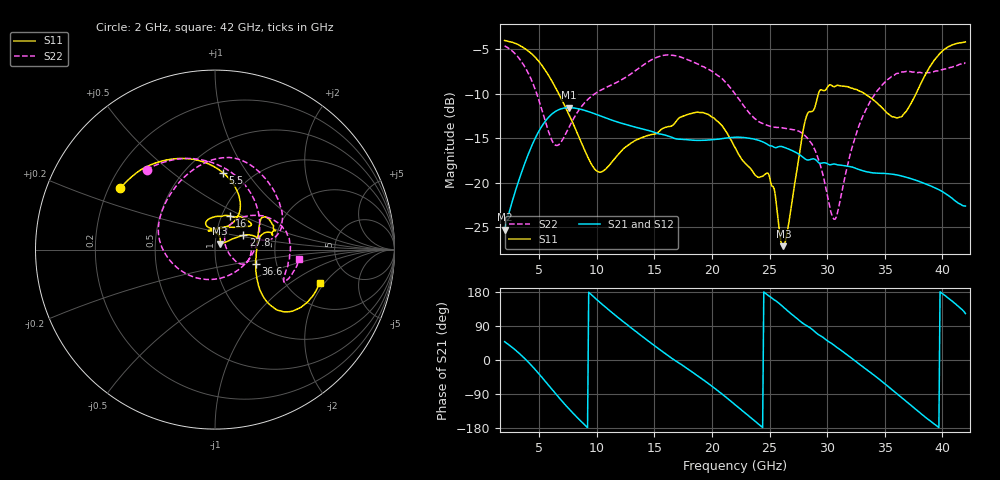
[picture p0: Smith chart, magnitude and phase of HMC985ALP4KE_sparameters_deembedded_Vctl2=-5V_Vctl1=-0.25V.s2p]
!s2p File: Measurements: S11, S21, S12, S22
# GHz S dB R 50.0
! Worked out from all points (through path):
!   401 points, 2 GHz to 42 GHz, reference 50 ohm
!   highest |S21| = -11.58 dB at 7.6 GHz (marker M1); lowest = -25.3 dB at 2 GHz (marker M2)
!   lowest |S11| = -27.1 dB at 26.2 GHz (marker M3), VSWR 1.09, Z = 52.8 + j3.54 ohm
!   |S11| at or under -10 dB: 6.69 GHz to 29.25 GHz (22.56 GHz wide, 126 % of centre); 33.24 GHz to 37.72 GHz (4.48 GHz wide, 12.6 % of centre)
!   |S22| runs from -24.1 to -4.6 dB; largest |S21 - S12| = 0.00027
!   S11 on the Smith chart (normalised r, x): 2 GHz: 0.25, +0.28; 5.5 GHz: 0.75, +0.78; 16 GHz: 1.09, +0.43; 27.8 GHz: 1.35, +0.22; 36.6 GHz: 1.56, -0.27; 42 GHz: 3.04, -1.80
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2  -4.04 147.2  -25.27 48.3  -25.27 48.3  -4.64 130.6
3.6  -4.83 120.5  -18.36 8.2  -18.36 8.2  -6.68 85.2
5.5  -7.33 84.0  -13.16 -55.2  -13.16 -55.2  -12.96 2.2
6.5  -9.53 66.9  -11.93 -91.5  -11.94 -91.5  -15.82 -70.7
7.6  -12.39 56.2  -11.58 -129.4  -11.58 -129.4  -13.75 -137.2
8.7  -15.62 58.2  -11.79 -163.8  -11.80 -163.8  -11.41 -171.2
10.2  -18.79 86.9  -12.44 154.0  -12.45 154.0  -9.71 164.5
11.9  -16.78 110.0  -13.23 110.8  -13.24 110.9  -8.64 141.2
15.4  -14.26 76.4  -14.51 29.1  -14.52 29.1  -5.85 87.2
16  -13.77 66.5  -14.68 15.7  -14.68 15.7  -5.68 79.8
19.4  -12.21 34.3  -15.23 -55.7  -15.23 -55.7  -7.09 35.6
22  -16.04 52.0  -14.89 -117.7  -14.90 -117.7  -10.02 10.5
24.9  -18.98 103.2  -15.77 169.9  -15.78 169.9  -13.61 13.0
26.2  -27.11 49.2  -15.99 139.4  -16.00 139.4  -13.86 -1.7
27.8  -15.04 26.8  -17.03 99.0  -17.03 99.0  -14.41 -22.7
28.7  -12.00 12.6  -17.33 80.7  -17.34 80.8  -15.69 -29.2
30.7  -9.20 20.5  -17.91 36.6  -17.91 36.6  -24.07 23.0
32.9  -9.77 33.8  -18.58 -13.3  -18.59 -13.3  -13.15 52.2
35.4  -12.36 11.2  -19.00 -72.5  -19.00 -72.5  -8.29 21.8
36.6  -12.37 -19.4  -19.29 -102.9  -19.29 -102.8  -7.58 6.7
39.5  -5.95 -42.8  -20.65 -173.5  -20.65 -173.5  -7.46 -24.7
42  -4.21 -17.4  -22.61 122.6  -22.62 122.6  -6.52 -6.2
